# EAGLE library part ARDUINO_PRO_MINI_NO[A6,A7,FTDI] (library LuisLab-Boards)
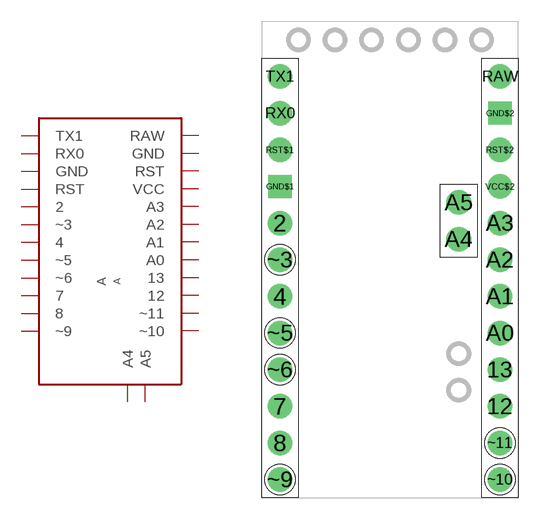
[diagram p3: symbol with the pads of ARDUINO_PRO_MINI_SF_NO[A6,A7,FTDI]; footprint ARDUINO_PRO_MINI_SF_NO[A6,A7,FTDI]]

Designator prefix A

## ARDUINO_PRO_MINI_NO[A6,A7,FTDI]  [ARDUINO_PRO_MINI_SF_NO[A6,A7,FTDI]]
2  2
4  4
7  7
8  8
12  12
13  13
A0  A0
A1  A1
A2  A2
A3  A3
A4  A4
A5  A5
GND$1  GND
GND$2  GND
RAW  RAW
RST$1  RST
RST$2  RST
RX0  RX0
TX1  TX1
VCC$2  VCC
~3  ~3
~5  ~5
~6  ~6
~9  ~9
~10  ~10
~11  ~11

## Footprint ARDUINO_PRO_MINI_SF_NO[A6,A7,FTDI] (pad centres in mm)
Arduino Pro Mini by SparkFun without A6, A7 and FTDI Serial TTL pads. Available in 5V and 3.3V versions.
drill 1.016 pad 1.7: 2 -7.62,2.54; 4 -7.62,-2.54; 7 -7.62,-10.16; 8 -7.62,-12.7; 12 7.62,-10.16; 13 7.62,-7.62; A0 7.62,-5.08; A1 7.62,-2.54; A2 7.62,0; A3 7.62,2.54; A4 4.763,1.429; A5 4.763,3.969; RAW 7.62,12.7; RST$1 -7.62,7.62; RST$2 7.62,7.62; RX0 -7.62,10.16; TX1 -7.62,12.7; VCC$2 7.62,5.08; ~3 -7.62,0; ~5 -7.62,-5.08; ~6 -7.62,-7.62; ~9 -7.62,-15.24; ~10 7.62,-15.24; ~11 7.62,-12.7
drill 1.016 pad 1.6 square: GND$1 -7.62,5.08; GND$2 7.62,10.16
